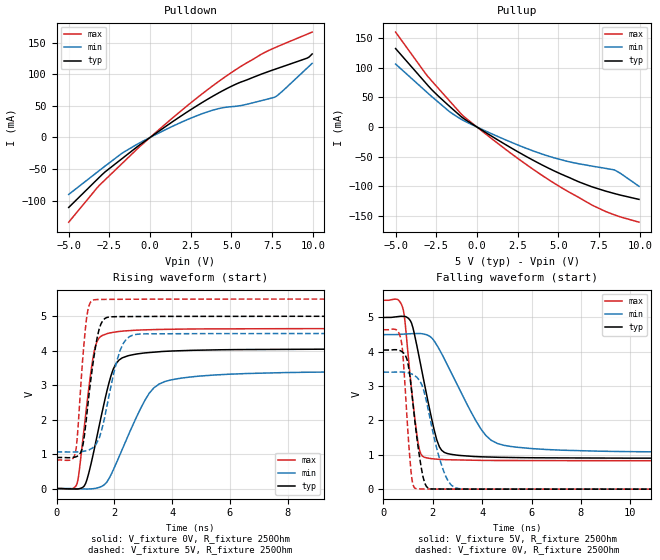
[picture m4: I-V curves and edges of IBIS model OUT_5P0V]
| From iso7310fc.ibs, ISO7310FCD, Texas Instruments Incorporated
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|   Model OUT_5P0V
[Model]   OUT_5P0V
Model_type   Output
Polarity   Non-Inverting
Vmeas = 2.5
Vref = 2.5
Cref = 15pF
Rref = 250
|   typ   min   max
|   (nom PVT)   (slow PVT)   (fast PVT)
C_comp   0.693p   0.662p   0.695p
|C_comp (ON state)   0.720p   0.656p   0.724p
|C_comp (OFF state)   0.693p   0.662p   0.695p
| Where   nom PVT is  Nominal Process, 5.0V, 27C
|   Fast PVT is Strong Process, 5.5V, -40C
|   Slow PVT is Weak Process, 4.5V, 150C
[Voltage Range]   5   4.5   5.5
[Temperature Range]   27   150   -40
[Pullup Reference]   5   4.5   5.5
[Pulldown Reference]   0   0   0
[Power Clamp Reference]   5   4.5   5.5
[GND Clamp Reference]   0   0   0
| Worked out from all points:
|   slope of the pulldown table from 0 to 0.75 V, typ, clamps not added: 54.8 ohm
|   slope of the pullup table from 0 to 0.75 V, typ, clamps not added: 58.4 ohm
|   falling waveform, V_fixture 5V, R_fixture 250Ohm: 20-80 % time 703ps typ, 1.5ns min, 408ps max; typ from 5 V to 0.903 V
|   rising waveform, V_fixture 0V, R_fixture 250Ohm: 20-80 % time 653ps typ, 1.14ns min, 402ps max; typ from 0 V to 4.05 V
|   rising waveform, V_fixture 5V, R_fixture 250Ohm: 20-80 % time 373ps typ, 549ps min, 247ps max; typ from 0.901 V to 5 V
|   falling waveform, V_fixture 0V, R_fixture 250Ohm: 20-80 % time 412ps typ, 679ps min, 258ps max; typ from 4.05 V to 0 V
[Pulldown]
|   Voltage   I(typ)   I(min)   I(max)
-5V       -110.7mA   -90.12mA   -134mA
-3.125V   -63.2mA    -52.44mA   -75.92mA
-1.705V   -33.12mA   -24.6mA    -40.78mA
-635mV    -11.7mA    -8.5mA     -14.38mA
805mV     14.68mA    10.51mA    18.15mA
3.115V    53.95mA    36.75mA    67.31mA
4.315V    71.91mA    46.26mA    90.48mA
5.185V    83.3mA     49.09mA    105.9mA
6.82V     100mA      58.13mA    131.5mA
7.69V     108mA      64.14mA    142.2mA
9.655V    125.6mA    110mA      163.5mA
9.955V    132.1mA    117.2mA    166.7mA
[Pullup]
|   Voltage   I(typ)   I(min)   I(max)
-5V       131.9mA    105.9mA    159.6mA
-3.125V   73.33mA    59.68mA    88.62mA
-2.765V   62.41mA    50.9mA     77.08mA
-1.705V   35.3mA     26.21mA    44.53mA
-965mV    17.33mA    13mA       21.8mA
805mV     -13.77mA   -10.11mA   -17.44mA
3.4V      -55.11mA   -39.63mA   -70.14mA
4.42V     -69.52mA   -49.18mA   -88.84mA
5.575V    -83.89mA   -57.87mA   -108.1mA
7.135V    -101.2mA   -66.04mA   -132.2mA
8.44V     -111.8mA   -72.11mA   -147.7mA
9.955V    -121.6mA   -99.65mA   -160mA
[Ramp]
R_load = 250
|   typ   min   max
dV/dt_r   2.42854/6.53221e-10   2.04442/1.14007e-09   2.78516/4.02068e-10
dV/dt_f   2.458/7.03353e-10   2.06133/1.49589e-09   2.80253/4.07617e-10
[Falling Waveform]
V_fixture = 5V
V_fixture_min = 4.5V
V_fixture_max = 5.5V
R_fixture = 250Ohm
C_fixture = 0F
|   Time   V(typ)   V(min)   V(max)
0s        5V         4.5V       5.5V
794.1ps   5.032V     4.513V     5.252V
1.14ns    4.833V     4.528V     2.915V
1.41ns    3.981V     4.531V     1.324V
1.692ns   2.959V     4.507V     922.2mV
2.159ns   1.439V     4.2V       873.2mV
2.361ns   1.13V      3.942V     865mV
3.943ns   942.9mV    1.759V     838.8mV
4.905ns   925.3mV    1.274V     834.7mV
19.9ns    903.3mV    1.064V     829.1mV
[Rising Waveform]
V_fixture = 0V
V_fixture_min = 0V
V_fixture_max = 0V
R_fixture = 250Ohm
C_fixture = 0F
|   Time   V(typ)   V(min)   V(max)
0s        908.5pV    4.27nV     840.3pV
708.8ps   -15.22mV   -6.496mV   137.5mV
1.009ns   152.2mV    -13.38mV   2.148V
1.315ns   1.177V     746.8uV    4.03V
1.758ns   2.874V     208.5mV    4.498V
1.959ns   3.457V     531.4mV    4.535V
2.27ns    3.792V     1.128V     4.568V
3.21ns    3.947V     2.767V     4.61V
3.943ns   3.99V      3.149V     4.623V
19.9ns    4.048V     3.407V     4.642V
[Rising Waveform]
V_fixture = 5V
V_fixture_min = 4.5V
V_fixture_max = 5.5V
R_fixture = 250Ohm
C_fixture = 0F
|   Time   V(typ)   V(min)   V(max)
0s        900.7mV    1.062V     829.1mV
653.7ps   916.1mV    1.061V     1.037V
739.5ps   950.1mV    1.064V     1.717V
882.3ps   1.146V     1.076V     3.491V
1.034ns   2.041V     1.099V     4.909V
1.276ns   3.713V     1.202V     5.473V
1.603ns   4.876V     1.833V     5.49V
2.207ns   4.991V     4.022V     5.493V
2.762ns   4.993V     4.475V     5.496V
19.9ns    5V         4.5V       5.5V
[Falling Waveform]
|Gnd
V_fixture = 0V
V_fixture_min = 0V
V_fixture_max = 0V
R_fixture = 250Ohm
C_fixture = 0F
|   Time   V(typ)   V(min)   V(max)
0s        4.051V     3.408V     4.642V
708.8ps   4.022V     3.411V     4.367V
794.1ps   3.978V     3.409V     3.868V
961.3ps   3.763V     3.394V     2.018V
1.122ns   2.983V     3.36V      495.1mV
1.315ns   1.731V     3.279V     16.01mV
1.742ns   78.06mV    2.56V      4.036mV
2.419ns   3.526mV    565.5mV    2.63mV
3.06ns    2.628mV    14.93mV    1.453mV
19.9ns    143.5uV    46uV       43.1uV
